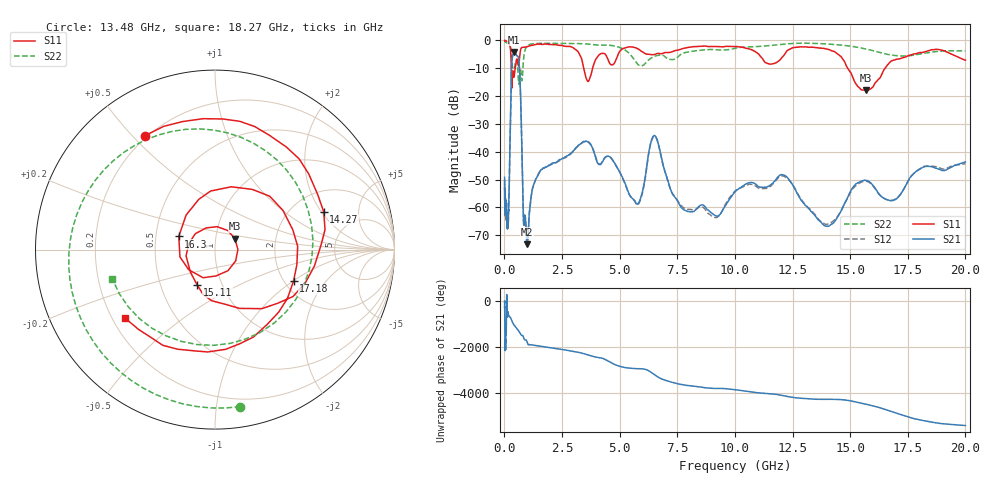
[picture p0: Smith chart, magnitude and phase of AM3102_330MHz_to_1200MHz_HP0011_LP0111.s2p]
! Date/Time: Tue, Sep 11, 2018 5:12 PM
! Network Analyzer: Agilent Technologies E8362B Rev: A.07.50.63
! Sweep from 0.010 to 20.000 GHz, 1601 Points, Sweep Type: LOG
! Power Supply: 4.950 V, 0.001 A
# Hz S DB R 50
!freq MagS11 AngS11 MagS21 AngS21 MagS12 AngS12 MagS22 AngS22
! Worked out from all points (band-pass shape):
!   1601 points, 10 MHz to 20 GHz, reference 50 ohm
!   highest |S21| = -4.16 dB at 424.4 MHz (marker M1); lowest = -73.3 dB at 988.7 MHz (marker M2)
!   |S21| within 3 dB of the highest: 329.7 MHz to 626.9 MHz (297.2 MHz wide, 62.1 % of centre)
!   lowest |S11| = -18.0 dB at 15.7 GHz (marker M3), VSWR 1.29, Z = 62 + j7.65 ohm
!   |S11| at or under -10 dB: 298.5 MHz to 468.5 MHz (170 MHz wide, 44.3 % of centre); 3.442 GHz to 3.826 GHz (383.8 MHz wide, 10.6 % of centre); 14.89 GHz to 16.51 GHz (1.62 GHz wide, 10.3 % of centre)
!   |S22| runs from -15.7 to -0.2 dB; largest |S21 - S12| = 0.01
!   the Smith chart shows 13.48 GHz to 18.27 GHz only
!   S11 on the Smith chart (normalised r, x): 13.48 GHz: 0.19, +0.54; 14.27 GHz: 2.95, +2.11; 15.11 GHz: 0.76, -0.31; 16.3 GHz: 0.66, +0.10; 17.18 GHz: 2.24, -1.01; 18.27 GHz: 0.25, -0.32
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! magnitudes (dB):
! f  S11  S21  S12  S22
! 10 MHz  0.0  -49.2  -53.6  -0.2
! 35.55 MHz  0.0  -60.5  -62.3  -0.4
! 126.4 MHz  -0.4  -66.9  -64.2  -1.0
! 179.6 MHz  -0.9  -61.8  -63.1  -1.2
! 424.4 MHz  -12.9  -4.2  -4.2  -10.2
! 447.2 MHz  -11.2  -4.3  -4.3  -9.0
! 650.9 MHz  -6.9  -9.6  -9.6  -13.9
! 833.3 MHz  -2.4  -65.3  -65.8  -6.6
! 988.7 MHz  -2.2  -73.3  -73.9  -2.0
! 1.59 GHz  -1.4  -46.5  -46.6  -1.0
! 3.582 GHz  -14.2  -36.3  -36.2  -1.3
! 5.652 GHz  -2.5  -57.6  -57.8  -7.1
! 6.518 GHz  -5.0  -34.2  -34.4  -5.7
! 7.882 GHz  -2.7  -61.3  -60.5  -4.3
! 13.48 GHz  -2.6  -63.0  -62.6  -1.0
! 14.27 GHz  -3.9  -65.7  -64.8  -1.4
! 15.11 GHz  -13.2  -52.9  -53.4  -2.2
! 15.7 GHz  -18.0  -50.3  -50.6  -3.1
! 16.3 GHz  -13.4  -55.7  -55.7  -4.3
! 17.18 GHz  -6.5  -55.5  -55.3  -5.6
! 18.27 GHz  -4.0  -45.3  -45.2  -4.5
! 20 GHz  -7.1  -43.7  -44.3  -3.7
